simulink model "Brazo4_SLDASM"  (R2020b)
settings: Solver=VariableStepAuto  StartTime=0.0  StopTime=20  RelTol=1e-3
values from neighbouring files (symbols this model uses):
  q = [q 0]    [robotSimulation.m]    (also in robotSimulationWithConstraints.m = [q' 0])
undefined symbols (not defined in the file or in its folder): deg, kg, m, N, rad, s, X, Y, Z
libraries: sm_lib x118, nesl_utility x17, pid_lib x4
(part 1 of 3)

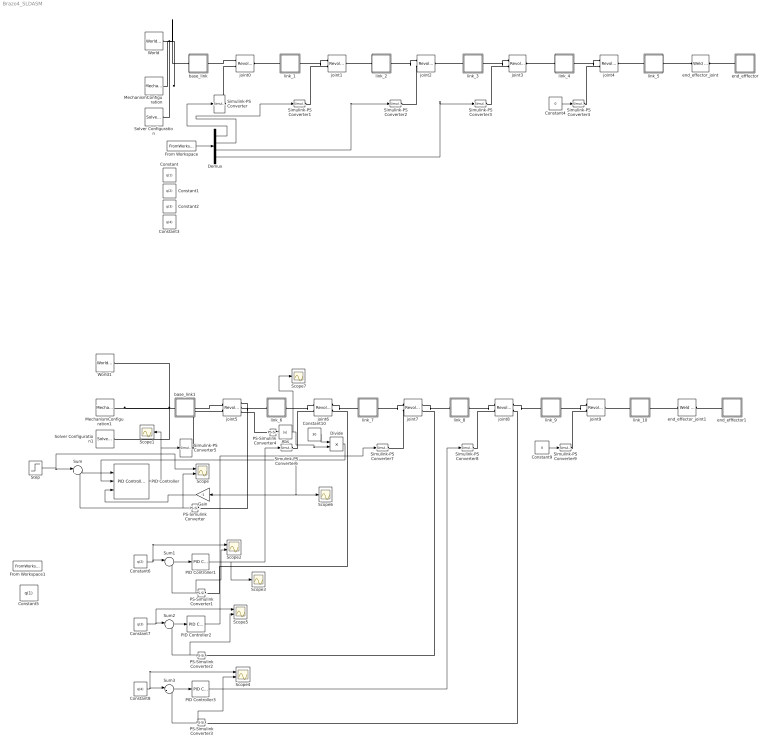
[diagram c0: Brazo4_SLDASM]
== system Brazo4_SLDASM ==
  Abs : Abs
  Constant : Constant  Commented=on  Value=q(1)
  Constant1 : Constant  Commented=on  Value=q(2)
  Constant10 : Constant  Value=30
  Constant2 : Constant  Commented=on  Value=q(3)
  Constant3 : Constant  Commented=on  Value=q(4)
  Constant4 : Constant  Commented=on  Value=0
  Constant5 : Constant  Value=q(1)
  Constant6 : Constant  Value=q(2)
  Constant7 : Constant  Value=q(3)
  Constant8 : Constant  Value=q(4)
  Constant9 : Constant  Value=0
  Demux : Demux  Commented=on
  Divide : Product  Inputs=*/
  From Workspace : FromWorkspace  Commented=on  VariableName=simq
  From Workspace1 : FromWorkspace  VariableName=simq
  Gain : Gain  Gain=-1
  MechanismConfiguration : sm_lib/Utilities/Mechanism Configuration  Commented=on  UniformGravity=Constant  GravityVector=[0 0 -9.80665]  GravityVectorUnits=m/s^2  GravityUnits=m/s^2  LinearizationDelta=0.001  JointModeTransitionNonlinearIterations=2
  MechanismConfiguration1 : sm_lib/Utilities/Mechanism Configuration  UniformGravity=Constant  GravityVector=[0 0 -9.80665]  GravityVectorUnits=m/s^2  GravityUnits=m/s^2  LinearizationDelta=0.001  JointModeTransitionNonlinearIterations=2
  PID Controller : pid_lib/PID Controller  Controller=PD  Form=Parallel  TimeDomain=Continuous-time  UseExternalTs=off  SampleTime=-1  IntegratorMethod=Forward Euler  FilterMethod=Forward Euler  ControllerParametersSource=internal  P=28.6165080032906  I=470.75049682787  D=20.8749963789507  UseFilter=on  N=748.537517356487  TunerSelectOption=Transfer Function Based (PID Tuner App)  InitialConditionSource=internal  InitialConditionForIntegrator=0  InitialConditionForFilter=0  DifferentiatorICPrevScaledInput=0  ExternalReset=none  TrackingMode=off  Kt=1  LimitOutput=on  SatLimitsSource=external  UpperSaturationLimit=inf  LowerSaturationLimit=-inf  LinearizeAsGain=on  AntiWindupMode=none  Kb=1  POutMin=[]  POutMax=[]  IOutMin=[]  IOutMax=[]  DOutMin=[]  DOutMax=[]  NOutMin=[]  NOutMax=[]  SumOutMin=[]  SumOutMax=[]  SaturationOutMin=[]  SaturationOutMax=[]  PParamMin=[]  PParamMax=[]  IParamMin=[]  IParamMax=[]  DParamMin=[]  DParamMax=[]  NParamMin=[]  NParamMax=[]  KbParamMin=[]  KbParamMax=[]  KtParamMin=[]  KtParamMax=[]  KbOutMin=[]  KbOutMax=[]  KtOutMin=[]  KtOutMax=[]  IntegratorOutMin=[]  IntegratorOutMax=[]  FilterOutMin=[]  FilterOutMax=[]  SumI1OutMin=[]  SumI1OutMax=[]  SumI2OutMin=[]  SumI2OutMax=[]  SumI3OutMin=[]  SumI3OutMax=[]  SumI4OutMin=[]  SumI4OutMax=[]  SumDOutMin=[]  SumDOutMax=[]  DifferentiatorOutMin=[]  DifferentiatorOutMax=[]  FilterDiffOutCoefMin=[]  FilterDiffOutCoefMax=[]  ReciprocalOutMin=[]  ReciprocalOutMax=[]  SumDenOutMin=[]  SumDenOutMax=[]  SumNumOutMin=[]  SumNumOutMax=[]  DivideOutMin=[]  DivideOutMax=[]  UdiffTsProdOutMin=[]  UdiffTsProdOutMax=[]  NTsProdOutMin=[]  NTsProdOutMax=[]  UintegralTsProdOutMin=[]  UintegralTsProdOutMax=[]  UngainTsProdOutMin=[]  UngainTsProdOutMax=[]  IntegratorContinuousStateAttributes=''  IntegratorStateMustResolveToSignalObject=off  IntegratorRTWStateStorageClass=Auto  FilterContinuousStateAttributes=''  FilterStateMustResolveToSignalObject=off  FilterRTWStateStorageClass=Auto  ParallelPVariant=InternalParameters  IdealPVariant=Disabled  IVariant=Disabled  DVariant=InternalParameters  IntegratorVariant=Disabled  SatVariant=External  AWVariant=Disabled  PCopyVariant=Disabled  TRVariant=Disabled  FdbkBlocksVariant=Forward  IdealPFdbkVariant=Disabled  SatFdbkVariant=Disabled  DerivativeFilterVariant=ContFilter  NVariant=InternalParameters  NCopyVariant=Disabled  FilterICVariant=InternalICsFilter  IntegratorICVariant=Disabled  ExternalResetVariant=Disabled  TRSumVariant=Passthrough  SumFdbkVariant=Disabled  SumVariant=Sum_PD  TsampFilterVariant=InternalTs  TsampNgainVariant=Passthrough  TsampIntegralVariant=Disabled_SignalSpec  ExternalSaturationOutDataTypeStr=Inherit: Same as second input
  PID Controller1 : pid_lib/PID Controller  Controller=PID  Form=Parallel  TimeDomain=Continuous-time  UseExternalTs=off  SampleTime=-1  IntegratorMethod=Forward Euler  FilterMethod=Forward Euler  ControllerParametersSource=internal  P=623.560595989225  I=560.575968398352  D=154.114613829274  UseFilter=on  N=17610.6564225781  TunerSelectOption=Transfer Function Based (PID Tuner App)  InitialConditionSource=internal  InitialConditionForIntegrator=0  InitialConditionForFilter=0  DifferentiatorICPrevScaledInput=0  ExternalReset=none  TrackingMode=off  Kt=1  LimitOutput=off  SatLimitsSource=internal  UpperSaturationLimit=inf  LowerSaturationLimit=-inf  LinearizeAsGain=on  AntiWindupMode=none  Kb=1  POutMin=[]  POutMax=[]  IOutMin=[]  IOutMax=[]  DOutMin=[]  DOutMax=[]  NOutMin=[]  NOutMax=[]  SumOutMin=[]  SumOutMax=[]  SaturationOutMin=[]  SaturationOutMax=[]  PParamMin=[]  PParamMax=[]  IParamMin=[]  IParamMax=[]  DParamMin=[]  DParamMax=[]  NParamMin=[]  NParamMax=[]  KbParamMin=[]  KbParamMax=[]  KtParamMin=[]  KtParamMax=[]  KbOutMin=[]  KbOutMax=[]  KtOutMin=[]  KtOutMax=[]  IntegratorOutMin=[]  IntegratorOutMax=[]  FilterOutMin=[]  FilterOutMax=[]  SumI1OutMin=[]  SumI1OutMax=[]  SumI2OutMin=[]  SumI2OutMax=[]  SumI3OutMin=[]  SumI3OutMax=[]  SumI4OutMin=[]  SumI4OutMax=[]  SumDOutMin=[]  SumDOutMax=[]  DifferentiatorOutMin=[]  DifferentiatorOutMax=[]  FilterDiffOutCoefMin=[]  FilterDiffOutCoefMax=[]  ReciprocalOutMin=[]  ReciprocalOutMax=[]  SumDenOutMin=[]  SumDenOutMax=[]  SumNumOutMin=[]  SumNumOutMax=[]  DivideOutMin=[]  DivideOutMax=[]  UdiffTsProdOutMin=[]  UdiffTsProdOutMax=[]  NTsProdOutMin=[]  NTsProdOutMax=[]  UintegralTsProdOutMin=[]  UintegralTsProdOutMax=[]  UngainTsProdOutMin=[]  UngainTsProdOutMax=[]  IntegratorContinuousStateAttributes=''  IntegratorStateMustResolveToSignalObject=off  IntegratorRTWStateStorageClass=Auto  FilterContinuousStateAttributes=''  FilterStateMustResolveToSignalObject=off  FilterRTWStateStorageClass=Auto  ParallelPVariant=InternalParameters  IdealPVariant=Disabled  IVariant=InternalParameters  DVariant=InternalParameters  IntegratorVariant=Continuous  SatVariant=Disabled  AWVariant=Passthrough  PCopyVariant=Disabled  TRVariant=Disabled  FdbkBlocksVariant=Forward  IdealPFdbkVariant=Disabled  SatFdbkVariant=Disabled  DerivativeFilterVariant=ContFilter  NVariant=InternalParameters  NCopyVariant=Disabled  FilterICVariant=InternalICsFilter  IntegratorICVariant=InternalICs  ExternalResetVariant=Disabled  TRSumVariant=Passthrough  SumFdbkVariant=Disabled  SumVariant=Sum_PID  TsampFilterVariant=InternalTs  TsampNgainVariant=Passthrough  TsampIntegralVariant=Passthrough  ExternalSaturationOutDataTypeStr=Inherit: Same as second input
  PID Controller2 : pid_lib/PID Controller  Controller=PID  Form=Parallel  TimeDomain=Continuous-time  UseExternalTs=off  SampleTime=-1  IntegratorMethod=Forward Euler  FilterMethod=Forward Euler  ControllerParametersSource=internal  P=25.434810287757  I=25.1632228084928  D=5.35733231569528  UseFilter=on  N=32.4755687633338  TunerSelectOption=Transfer Function Based (PID Tuner App)  InitialConditionSource=internal  InitialConditionForIntegrator=0  InitialConditionForFilter=0  DifferentiatorICPrevScaledInput=0  ExternalReset=none  TrackingMode=off  Kt=1  LimitOutput=off  SatLimitsSource=internal  UpperSaturationLimit=inf  LowerSaturationLimit=-inf  LinearizeAsGain=on  AntiWindupMode=none  Kb=1  POutMin=[]  POutMax=[]  IOutMin=[]  IOutMax=[]  DOutMin=[]  DOutMax=[]  NOutMin=[]  NOutMax=[]  SumOutMin=[]  SumOutMax=[]  SaturationOutMin=[]  SaturationOutMax=[]  PParamMin=[]  PParamMax=[]  IParamMin=[]  IParamMax=[]  DParamMin=[]  DParamMax=[]  NParamMin=[]  NParamMax=[]  KbParamMin=[]  KbParamMax=[]  KtParamMin=[]  KtParamMax=[]  KbOutMin=[]  KbOutMax=[]  KtOutMin=[]  KtOutMax=[]  IntegratorOutMin=[]  IntegratorOutMax=[]  FilterOutMin=[]  FilterOutMax=[]  SumI1OutMin=[]  SumI1OutMax=[]  SumI2OutMin=[]  SumI2OutMax=[]  SumI3OutMin=[]  SumI3OutMax=[]  SumI4OutMin=[]  SumI4OutMax=[]  SumDOutMin=[]  SumDOutMax=[]  DifferentiatorOutMin=[]  DifferentiatorOutMax=[]  FilterDiffOutCoefMin=[]  FilterDiffOutCoefMax=[]  ReciprocalOutMin=[]  ReciprocalOutMax=[]  SumDenOutMin=[]  SumDenOutMax=[]  SumNumOutMin=[]  SumNumOutMax=[]  DivideOutMin=[]  DivideOutMax=[]  UdiffTsProdOutMin=[]  UdiffTsProdOutMax=[]  NTsProdOutMin=[]  NTsProdOutMax=[]  UintegralTsProdOutMin=[]  UintegralTsProdOutMax=[]  UngainTsProdOutMin=[]  UngainTsProdOutMax=[]  IntegratorContinuousStateAttributes=''  IntegratorStateMustResolveToSignalObject=off  IntegratorRTWStateStorageClass=Auto  FilterContinuousStateAttributes=''  FilterStateMustResolveToSignalObject=off  FilterRTWStateStorageClass=Auto  ParallelPVariant=InternalParameters  IdealPVariant=Disabled  IVariant=InternalParameters  DVariant=InternalParameters  IntegratorVariant=Continuous  SatVariant=Disabled  AWVariant=Passthrough  PCopyVariant=Disabled  TRVariant=Disabled  FdbkBlocksVariant=Forward  IdealPFdbkVariant=Disabled  SatFdbkVariant=Disabled  DerivativeFilterVariant=ContFilter  NVariant=InternalParameters  NCopyVariant=Disabled  FilterICVariant=InternalICsFilter  IntegratorICVariant=InternalICs  ExternalResetVariant=Disabled  TRSumVariant=Passthrough  SumFdbkVariant=Disabled  SumVariant=Sum_PID  TsampFilterVariant=InternalTs  TsampNgainVariant=Passthrough  TsampIntegralVariant=Passthrough  ExternalSaturationOutDataTypeStr=Inherit: Same as second input
  PID Controller3 : pid_lib/PID Controller  Controller=PID  Form=Parallel  TimeDomain=Continuous-time  UseExternalTs=off  SampleTime=-1  IntegratorMethod=Forward Euler  FilterMethod=Forward Euler  ControllerParametersSource=internal  P=5.46250972225863  I=4.50861619061035  D=1.47049025552506  UseFilter=on  N=16168.5388750867  TunerSelectOption=Transfer Function Based (PID Tuner App)  InitialConditionSource=internal  InitialConditionForIntegrator=0  InitialConditionForFilter=0  DifferentiatorICPrevScaledInput=0  ExternalReset=none  TrackingMode=off  Kt=1  LimitOutput=off  SatLimitsSource=internal  UpperSaturationLimit=inf  LowerSaturationLimit=-inf  LinearizeAsGain=on  AntiWindupMode=none  Kb=1  POutMin=[]  POutMax=[]  IOutMin=[]  IOutMax=[]  DOutMin=[]  DOutMax=[]  NOutMin=[]  NOutMax=[]  SumOutMin=[]  SumOutMax=[]  SaturationOutMin=[]  SaturationOutMax=[]  PParamMin=[]  PParamMax=[]  IParamMin=[]  IParamMax=[]  DParamMin=[]  DParamMax=[]  NParamMin=[]  NParamMax=[]  KbParamMin=[]  KbParamMax=[]  KtParamMin=[]  KtParamMax=[]  KbOutMin=[]  KbOutMax=[]  KtOutMin=[]  KtOutMax=[]  IntegratorOutMin=[]  IntegratorOutMax=[]  FilterOutMin=[]  FilterOutMax=[]  SumI1OutMin=[]  SumI1OutMax=[]  SumI2OutMin=[]  SumI2OutMax=[]  SumI3OutMin=[]  SumI3OutMax=[]  SumI4OutMin=[]  SumI4OutMax=[]  SumDOutMin=[]  SumDOutMax=[]  DifferentiatorOutMin=[]  DifferentiatorOutMax=[]  FilterDiffOutCoefMin=[]  FilterDiffOutCoefMax=[]  ReciprocalOutMin=[]  ReciprocalOutMax=[]  SumDenOutMin=[]  SumDenOutMax=[]  SumNumOutMin=[]  SumNumOutMax=[]  DivideOutMin=[]  DivideOutMax=[]  UdiffTsProdOutMin=[]  UdiffTsProdOutMax=[]  NTsProdOutMin=[]  NTsProdOutMax=[]  UintegralTsProdOutMin=[]  UintegralTsProdOutMax=[]  UngainTsProdOutMin=[]  UngainTsProdOutMax=[]  IntegratorContinuousStateAttributes=''  IntegratorStateMustResolveToSignalObject=off  IntegratorRTWStateStorageClass=Auto  FilterContinuousStateAttributes=''  FilterStateMustResolveToSignalObject=off  FilterRTWStateStorageClass=Auto  ParallelPVariant=InternalParameters  IdealPVariant=Disabled  IVariant=InternalParameters  DVariant=InternalParameters  IntegratorVariant=Continuous  SatVariant=Disabled  AWVariant=Passthrough  PCopyVariant=Disabled  TRVariant=Disabled  FdbkBlocksVariant=Forward  IdealPFdbkVariant=Disabled  SatFdbkVariant=Disabled  DerivativeFilterVariant=ContFilter  NVariant=InternalParameters  NCopyVariant=Disabled  FilterICVariant=InternalICsFilter  IntegratorICVariant=InternalICs  ExternalResetVariant=Disabled  TRSumVariant=Passthrough  SumFdbkVariant=Disabled  SumVariant=Sum_PID  TsampFilterVariant=InternalTs  TsampNgainVariant=Passthrough  TsampIntegralVariant=Passthrough  ExternalSaturationOutDataTypeStr=Inherit: Same as second input
  PS-Simulink Converter{,1..4} (5 alike) : nesl_utility/PS-Simulink Converter  PhysicalDomain=network_engine_domain  SubClassName=ps_output  LeftPortType=input  RightPortType=output  PseudoPeriodic=off  Frequencies=[]  Unit=inherit  AffineConversion=off
  Scope{,2,4..5} (4 alike) : Scope  NumInputPorts=2
  Scope{1,3,6..7} (4 alike) : Scope
  Simulink-PS Converter{,1..3} (4 alike) : nesl_utility/Simulink-PS Converter  Commented=on  PhysicalDomain=network_engine_domain  SubClassName=ps_input  LeftPortType=input  RightPortType=output  PseudoPeriodic=off  Frequencies=[]  NoiseDistribution=none  NoiseParameters=[]  Unit=1  AffineConversion=off  FilteringAndDerivatives=filter  SimscapeFilterOrder=2  InputFilterTimeConstant=0.001  UdotUserProvided=0
  Simulink-PS Converter4 : nesl_utility/Simulink-PS Converter  Commented=on  PhysicalDomain=network_engine_domain  SubClassName=ps_input  LeftPortType=input  RightPortType=output  PseudoPeriodic=off  Frequencies=[]  NoiseDistribution=none  NoiseParameters=[]  Unit=1  AffineConversion=off  FilteringAndDerivatives=provide  SimscapeFilterOrder=1  InputFilterTimeConstant=0.001  UdotUserProvided=0
  Simulink-PS Converter{5..8} (4 alike) : nesl_utility/Simulink-PS Converter  PhysicalDomain=network_engine_domain  SubClassName=ps_input  LeftPortType=input  RightPortType=output  PseudoPeriodic=off  Frequencies=[]  NoiseDistribution=none  NoiseParameters=[]  Unit=1  AffineConversion=off  FilteringAndDerivatives=filter  SimscapeFilterOrder=2  InputFilterTimeConstant=0.001  UdotUserProvided=0
  Simulink-PS Converter9 : nesl_utility/Simulink-PS Converter  PhysicalDomain=network_engine_domain  SubClassName=ps_input  LeftPortType=input  RightPortType=output  PseudoPeriodic=off  Frequencies=[]  NoiseDistribution=none  NoiseParameters=[]  Unit=1  AffineConversion=off  FilteringAndDerivatives=provide  SimscapeFilterOrder=1  InputFilterTimeConstant=0.001  UdotUserProvided=0
  Solver Configuration : nesl_utility/Solver Configuration  Commented=on  PhysicalDomain=network_engine_domain  SubClassName=solver  LeftPortType=input  RightPortType=generic  Tones=[]  Harmonics=[]  SimulateNoise=off  Profile=off  UseLocalSampling=off  EnableSwitchedLinearOptims=on  FrequencyDomain=off  UseCCode=off  RelTol=0.001  AbsTol=1e-06  MinStep=1e-09  ToWorkspace=off  RevertToSquareIcSolve=off  NumHomotopyIterations=100  PhasorMode=off  PhasorModeNumHarmonics=1  DoDC=off  ResidualTolerance=1e-09  UseLocalSolver=off  LocalSolverChoice=NE_BACKWARD_EULER_ADVANCER  LocalSolverSampleTime=0.001  DoFixedCost=off  MaxNonlinIter=3  MaxModeIter=2  ComputeImpulses=off  ImpulseIterations=2  LinearAlgebra=auto  EquationFormulation=NE_TIME_EF  DelaysMemoryBudget=1024  AutomaticFiltering=on  FilteringTimeConstant=0.001  PartitionStorageMethod=AS_NEEDED  PartitionMemoryBudget=1024  PartitionMethod=ROBUST
  Solver Configuration1 : nesl_utility/Solver Configuration  PhysicalDomain=network_engine_domain  SubClassName=solver  LeftPortType=input  RightPortType=generic  Tones=[]  Harmonics=[]  SimulateNoise=off  Profile=off  UseLocalSampling=off  EnableSwitchedLinearOptims=on  FrequencyDomain=off  UseCCode=off  RelTol=0.001  AbsTol=1e-06  MinStep=1e-09  ToWorkspace=off  RevertToSquareIcSolve=off  NumHomotopyIterations=100  PhasorMode=off  PhasorModeNumHarmonics=1  DoDC=off  ResidualTolerance=1e-09  UseLocalSolver=off  LocalSolverChoice=NE_BACKWARD_EULER_ADVANCER  LocalSolverSampleTime=0.001  DoFixedCost=off  MaxNonlinIter=3  MaxModeIter=2  ComputeImpulses=off  ImpulseIterations=2  LinearAlgebra=auto  EquationFormulation=NE_TIME_EF  DelaysMemoryBudget=1024  AutomaticFiltering=on  FilteringTimeConstant=0.001  PartitionStorageMethod=AS_NEEDED  PartitionMemoryBudget=1024  PartitionMethod=ROBUST
  Step : Step  After=q(1)  SampleTime=0
  Sum{,1..3} (4 alike) : Sum  Inputs=|+-
  World : sm_lib/Frames and Transforms/World Frame  Commented=on
  World1 : sm_lib/Frames and Transforms/World Frame
  base_link : Subsystem  Commented=on
  base_link1 : Subsystem
  end_effector_joint : sm_lib/Joints/Weld Joint  Commented=on  JointMode=Normal  SenseConstraintForce=off  SenseConstraintForceX=off  SenseConstraintForceY=off  SenseConstraintForceZ=off  SenseConstraintTorque=off  SenseConstraintTorqueX=off  SenseConstraintTorqueY=off  SenseConstraintTorqueZ=off  SenseTotalForce=off  SenseTotalForceX=off  SenseTotalForceY=off  SenseTotalForceZ=off  SenseTotalTorque=off  SenseTotalTorqueX=off  SenseTotalTorqueY=off  SenseTotalTorqueZ=off  CompositeWrenchDir=FollowerOnBase  CompositeWrenchFrame=BaseFrame
  end_effector_joint1 : sm_lib/Joints/Weld Joint  JointMode=Normal  SenseConstraintForce=off  SenseConstraintForceX=off  SenseConstraintForceY=off  SenseConstraintForceZ=off  SenseConstraintTorque=off  SenseConstraintTorqueX=off  SenseConstraintTorqueY=off  SenseConstraintTorqueZ=off  SenseTotalForce=off  SenseTotalForceX=off  SenseTotalForceY=off  SenseTotalForceZ=off  SenseTotalTorque=off  SenseTotalTorqueX=off  SenseTotalTorqueY=off  SenseTotalTorqueZ=off  CompositeWrenchDir=FollowerOnBase  CompositeWrenchFrame=BaseFrame
  end_efffector : Subsystem  Commented=on
  end_efffector1 : Subsystem
  joint0 : sm_lib/Joints/Revolute Joint  Commented=on  JointMode=Normal  SenseConstraintForce=off  SenseConstraintForceX=off  SenseConstraintForceY=off  SenseConstraintForceZ=off  SenseConstraintTorque=off  SenseConstraintTorqueX=off  SenseConstraintTorqueY=off  SenseConstraintTorqueZ=off  SenseTotalForce=off  SenseTotalForceX=off  SenseTotalForceY=off  SenseTotalForceZ=off  SenseTotalTorque=off  SenseTotalTorqueX=off  SenseTotalTorqueY=off  SenseTotalTorqueZ=off  CompositeWrenchDir=FollowerOnBase  CompositeWrenchFrame=BaseFrame  EquilibriumPosition=0  EquilibriumPositionUnits=deg  SpringStiffness=0  SpringStiffnessUnits=N*m/deg  DampingCoefficient=0  DampingCoefficientUnits=m^2*kg/s/rad  TorqueActuationMode=ComputedTorque  MotionActuationMode=InputMotion  SensePosition=off  SenseVelocity=off  SenseAcceleration=off  SenseTorqueForce=off  SenseLowerLimitTorqueForce=off  SenseUpperLimitTorqueForce=off  LowerLimitSpecify=on  LowerLimitBound=-2.618  LowerLimitBoundUnits=rad  LowerLimitStiffness=1e4  LowerLimitStiffnessUnits=N*m/deg  LowerLimitDamping=10  LowerLimitDampingUnits=N*m/(deg/s)  LowerLimitTransitionRegionWidth=0.1  LowerLimitTransitionRegionWidthUnits=deg  UpperLimitSpecify=on  UpperLimitBound=2.618  UpperLimitBoundUnits=rad  UpperLimitStiffness=1e4  UpperLimitStiffnessUnits=N*m/deg  UpperLimitDamping=10  UpperLimitDampingUnits=N*m/(deg/s)  UpperLimitTransitionRegionWidth=0.1  UpperLimitTransitionRegionWidthUnits=deg  PositionTargetSpecify=off  PositionTargetPriority=High  PositionTargetValue=0  PositionTargetValueUnits=deg  VelocityTargetSpecify=off  VelocityTargetPriority=High  VelocityTargetValue=0  VelocityTargetValueUnits=deg/s
  joint1 : sm_lib/Joints/Revolute Joint  Commented=on  JointMode=Normal  SenseConstraintForce=off  SenseConstraintForceX=off  SenseConstraintForceY=off  SenseConstraintForceZ=off  SenseConstraintTorque=off  SenseConstraintTorqueX=off  SenseConstraintTorqueY=off  SenseConstraintTorqueZ=off  SenseTotalForce=off  SenseTotalForceX=off  SenseTotalForceY=off  SenseTotalForceZ=off  SenseTotalTorque=off  SenseTotalTorqueX=off  SenseTotalTorqueY=off  SenseTotalTorqueZ=off  CompositeWrenchDir=FollowerOnBase  CompositeWrenchFrame=BaseFrame  EquilibriumPosition=0  EquilibriumPositionUnits=deg  SpringStiffness=0  SpringStiffnessUnits=N*m/deg  DampingCoefficient=0  DampingCoefficientUnits=m^2*kg/s/rad  TorqueActuationMode=ComputedTorque  MotionActuationMode=InputMotion  SensePosition=off  SenseVelocity=off  SenseAcceleration=off  SenseTorqueForce=off  SenseLowerLimitTorqueForce=off  SenseUpperLimitTorqueForce=off  LowerLimitSpecify=on  LowerLimitBound=-1.134  LowerLimitBoundUnits=rad  LowerLimitStiffness=1e4  LowerLimitStiffnessUnits=N*m/deg  LowerLimitDamping=10  LowerLimitDampingUnits=N*m/(deg/s)  LowerLimitTransitionRegionWidth=0.1  LowerLimitTransitionRegionWidthUnits=deg  UpperLimitSpecify=on  UpperLimitBound=1.134  UpperLimitBoundUnits=rad  UpperLimitStiffness=1e4  UpperLimitStiffnessUnits=N*m/deg  UpperLimitDamping=10  UpperLimitDampingUnits=N*m/(deg/s)  UpperLimitTransitionRegionWidth=0.1  UpperLimitTransitionRegionWidthUnits=deg  PositionTargetSpecify=off  PositionTargetPriority=High  PositionTargetValue=0  PositionTargetValueUnits=deg  VelocityTargetSpecify=off  VelocityTargetPriority=High  VelocityTargetValue=0  VelocityTargetValueUnits=deg/s
  joint2 : sm_lib/Joints/Revolute Joint  Commented=on  JointMode=Normal  SenseConstraintForce=off  SenseConstraintForceX=off  SenseConstraintForceY=off  SenseConstraintForceZ=off  SenseConstraintTorque=off  SenseConstraintTorqueX=off  SenseConstraintTorqueY=off  SenseConstraintTorqueZ=off  SenseTotalForce=off  SenseTotalForceX=off  SenseTotalForceY=off  SenseTotalForceZ=off  SenseTotalTorque=off  SenseTotalTorqueX=off  SenseTotalTorqueY=off  SenseTotalTorqueZ=off  CompositeWrenchDir=FollowerOnBase  CompositeWrenchFrame=BaseFrame  EquilibriumPosition=0  EquilibriumPositionUnits=deg  SpringStiffness=0  SpringStiffnessUnits=N*m/deg  DampingCoefficient=0  DampingCoefficientUnits=m^2*kg/s/rad  TorqueActuationMode=ComputedTorque  MotionActuationMode=InputMotion  SensePosition=off  SenseVelocity=off  SenseAcceleration=off  SenseTorqueForce=off  SenseLowerLimitTorqueForce=off  SenseUpperLimitTorqueForce=off  LowerLimitSpecify=on  LowerLimitBound=-0.96  LowerLimitBoundUnits=rad  LowerLimitStiffness=1e4  LowerLimitStiffnessUnits=N*m/deg  LowerLimitDamping=10  LowerLimitDampingUnits=N*m/(deg/s)  LowerLimitTransitionRegionWidth=0.1  LowerLimitTransitionRegionWidthUnits=deg  UpperLimitSpecify=on  UpperLimitBound=0.96  UpperLimitBoundUnits=rad  UpperLimitStiffness=1e4  UpperLimitStiffnessUnits=N*m/deg  UpperLimitDamping=10  UpperLimitDampingUnits=N*m/(deg/s)  UpperLimitTransitionRegionWidth=0.1  UpperLimitTransitionRegionWidthUnits=deg  PositionTargetSpecify=off  PositionTargetPriority=High  PositionTargetValue=0  PositionTargetValueUnits=deg  VelocityTargetSpecify=off  VelocityTargetPriority=High  VelocityTargetValue=0  VelocityTargetValueUnits=deg/s
  joint3 : sm_lib/Joints/Revolute Joint  Commented=on  JointMode=Normal  SenseConstraintForce=off  SenseConstraintForceX=off  SenseConstraintForceY=off  SenseConstraintForceZ=off  SenseConstraintTorque=off  SenseConstraintTorqueX=off  SenseConstraintTorqueY=off  SenseConstraintTorqueZ=off  SenseTotalForce=off  SenseTotalForceX=off  SenseTotalForceY=off  SenseTotalForceZ=off  SenseTotalTorque=off  SenseTotalTorqueX=off  SenseTotalTorqueY=off  SenseTotalTorqueZ=off  CompositeWrenchDir=FollowerOnBase  CompositeWrenchFrame=BaseFrame  EquilibriumPosition=0  EquilibriumPositionUnits=deg  SpringStiffness=0  SpringStiffnessUnits=N*m/deg  DampingCoefficient=0  DampingCoefficientUnits=m^2*kg/s/rad  TorqueActuationMode=ComputedTorque  MotionActuationMode=InputMotion  SensePosition=off  SenseVelocity=off  SenseAcceleration=off  SenseTorqueForce=off  SenseLowerLimitTorqueForce=off  SenseUpperLimitTorqueForce=off  LowerLimitSpecify=on  LowerLimitBound=-1.57  LowerLimitBoundUnits=rad  LowerLimitStiffness=1e4  LowerLimitStiffnessUnits=N*m/deg  LowerLimitDamping=10  LowerLimitDampingUnits=N*m/(deg/s)  LowerLimitTransitionRegionWidth=0.1  LowerLimitTransitionRegionWidthUnits=deg  UpperLimitSpecify=on  UpperLimitBound=1.57  UpperLimitBoundUnits=rad  UpperLimitStiffness=1e4  UpperLimitStiffnessUnits=N*m/deg  UpperLimitDamping=10  UpperLimitDampingUnits=N*m/(deg/s)  UpperLimitTransitionRegionWidth=0.1  UpperLimitTransitionRegionWidthUnits=deg  PositionTargetSpecify=off  PositionTargetPriority=High  PositionTargetValue=0  PositionTargetValueUnits=deg  VelocityTargetSpecify=off  VelocityTargetPriority=High  VelocityTargetValue=0  VelocityTargetValueUnits=deg/s
  joint4 : sm_lib/Joints/Revolute Joint  Commented=on  JointMode=Normal  SenseConstraintForce=off  SenseConstraintForceX=off  SenseConstraintForceY=off  SenseConstraintForceZ=off  SenseConstraintTorque=off  SenseConstraintTorqueX=off  SenseConstraintTorqueY=off  SenseConstraintTorqueZ=off  SenseTotalForce=off  SenseTotalForceX=off  SenseTotalForceY=off  SenseTotalForceZ=off  SenseTotalTorque=off  SenseTotalTorqueX=off  SenseTotalTorqueY=off  SenseTotalTorqueZ=off  CompositeWrenchDir=FollowerOnBase  CompositeWrenchFrame=BaseFrame  EquilibriumPosition=0  EquilibriumPositionUnits=deg  SpringStiffness=0  SpringStiffnessUnits=N*m/deg  DampingCoefficient=0  DampingCoefficientUnits=m^2*kg/s/rad  TorqueActuationMode=ComputedTorque  MotionActuationMode=InputMotion  SensePosition=off  SenseVelocity=off  SenseAcceleration=off  SenseTorqueForce=off  SenseLowerLimitTorqueForce=off  SenseUpperLimitTorqueForce=off  LowerLimitSpecify=on  LowerLimitBound=-3.14  LowerLimitBoundUnits=rad  LowerLimitStiffness=1e4  LowerLimitStiffnessUnits=N*m/deg  LowerLimitDamping=10  LowerLimitDampingUnits=N*m/(deg/s)  LowerLimitTransitionRegionWidth=0.1  LowerLimitTransitionRegionWidthUnits=deg  UpperLimitSpecify=on  UpperLimitBound=3.14  UpperLimitBoundUnits=rad  UpperLimitStiffness=1e4  UpperLimitStiffnessUnits=N*m/deg  UpperLimitDamping=10  UpperLimitDampingUnits=N*m/(deg/s)  UpperLimitTransitionRegionWidth=0.1  UpperLimitTransitionRegionWidthUnits=deg  PositionTargetSpecify=off  PositionTargetPriority=High  PositionTargetValue=0  PositionTargetValueUnits=deg  VelocityTargetSpecify=off  VelocityTargetPriority=High  VelocityTargetValue=0  VelocityTargetValueUnits=deg/s
  joint5 : sm_lib/Joints/Revolute Joint  JointMode=Normal  SenseConstraintForce=off  SenseConstraintForceX=off  SenseConstraintForceY=off  SenseConstraintForceZ=off  SenseConstraintTorque=off  SenseConstraintTorqueX=off  SenseConstraintTorqueY=off  SenseConstraintTorqueZ=off  SenseTotalForce=off  SenseTotalForceX=off  SenseTotalForceY=off  SenseTotalForceZ=off  SenseTotalTorque=off  SenseTotalTorqueX=off  SenseTotalTorqueY=off  SenseTotalTorqueZ=off  CompositeWrenchDir=FollowerOnBase  CompositeWrenchFrame=BaseFrame  EquilibriumPosition=0  EquilibriumPositionUnits=deg  SpringStiffness=0  SpringStiffnessUnits=N*m/deg  DampingCoefficient=0  DampingCoefficientUnits=m^2*kg/s/rad  TorqueActuationMode=InputTorque  MotionActuationMode=ComputedMotion  SensePosition=on  SenseVelocity=on  SenseAcceleration=off  SenseTorqueForce=off  SenseLowerLimitTorqueForce=off  SenseUpperLimitTorqueForce=off  LowerLimitSpecify=on  LowerLimitBound=-2.618  LowerLimitBoundUnits=rad  LowerLimitStiffness=1e10  LowerLimitStiffnessUnits=N*m/deg  LowerLimitDamping=10000  LowerLimitDampingUnits=N*m/(deg/s)  LowerLimitTransitionRegionWidth=0.1  LowerLimitTransitionRegionWidthUnits=deg  UpperLimitSpecify=on  UpperLimitBound=2.618  UpperLimitBoundUnits=rad  UpperLimitStiffness=1e10  UpperLimitStiffnessUnits=N*m/deg  UpperLimitDamping=10000  UpperLimitDampingUnits=N*m/(deg/s)  UpperLimitTransitionRegionWidth=0.1  UpperLimitTransitionRegionWidthUnits=deg  PositionTargetSpecify=off  PositionTargetPriority=High  PositionTargetValue=0  PositionTargetValueUnits=deg  VelocityTargetSpecify=off  VelocityTargetPriority=High  VelocityTargetValue=0  VelocityTargetValueUnits=deg/s
  joint6 : sm_lib/Joints/Revolute Joint  JointMode=Normal  SenseConstraintForce=off  SenseConstraintForceX=off  SenseConstraintForceY=off  SenseConstraintForceZ=off  SenseConstraintTorque=off  SenseConstraintTorqueX=off  SenseConstraintTorqueY=off  SenseConstraintTorqueZ=off  SenseTotalForce=off  SenseTotalForceX=off  SenseTotalForceY=off  SenseTotalForceZ=off  SenseTotalTorque=off  SenseTotalTorqueX=off  SenseTotalTorqueY=off  SenseTotalTorqueZ=off  CompositeWrenchDir=FollowerOnBase  CompositeWrenchFrame=BaseFrame  EquilibriumPosition=0  EquilibriumPositionUnits=deg  SpringStiffness=0  SpringStiffnessUnits=N*m/deg  DampingCoefficient=0  DampingCoefficientUnits=m^2*kg/s/rad  TorqueActuationMode=InputTorque  MotionActuationMode=ComputedMotion  SensePosition=on  SenseVelocity=off  SenseAcceleration=off  SenseTorqueForce=off  SenseLowerLimitTorqueForce=off  SenseUpperLimitTorqueForce=off  LowerLimitSpecify=on  LowerLimitBound=-1.134  LowerLimitBoundUnits=rad  LowerLimitStiffness=1e4  LowerLimitStiffnessUnits=N*m/deg  LowerLimitDamping=10  LowerLimitDampingUnits=N*m/(deg/s)  LowerLimitTransitionRegionWidth=0.1  LowerLimitTransitionRegionWidthUnits=deg  UpperLimitSpecify=on  UpperLimitBound=1.134  UpperLimitBoundUnits=rad  UpperLimitStiffness=1e4  UpperLimitStiffnessUnits=N*m/deg  UpperLimitDamping=10  UpperLimitDampingUnits=N*m/(deg/s)  UpperLimitTransitionRegionWidth=0.1  UpperLimitTransitionRegionWidthUnits=deg  PositionTargetSpecify=off  PositionTargetPriority=High  PositionTargetValue=0  PositionTargetValueUnits=deg  VelocityTargetSpecify=off  VelocityTargetPriority=High  VelocityTargetValue=0  VelocityTargetValueUnits=deg/s
  joint7 : sm_lib/Joints/Revolute Joint  JointMode=Normal  SenseConstraintForce=off  SenseConstraintForceX=off  SenseConstraintForceY=off  SenseConstraintForceZ=off  SenseConstraintTorque=off  SenseConstraintTorqueX=off  SenseConstraintTorqueY=off  SenseConstraintTorqueZ=off  SenseTotalForce=off  SenseTotalForceX=off  SenseTotalForceY=off  SenseTotalForceZ=off  SenseTotalTorque=off  SenseTotalTorqueX=off  SenseTotalTorqueY=off  SenseTotalTorqueZ=off  CompositeWrenchDir=FollowerOnBase  CompositeWrenchFrame=BaseFrame  EquilibriumPosition=0  EquilibriumPositionUnits=deg  SpringStiffness=0  SpringStiffnessUnits=N*m/deg  DampingCoefficient=0  DampingCoefficientUnits=m^2*kg/s/rad  TorqueActuationMode=InputTorque  MotionActuationMode=ComputedMotion  SensePosition=on  SenseVelocity=off  SenseAcceleration=off  SenseTorqueForce=off  SenseLowerLimitTorqueForce=off  SenseUpperLimitTorqueForce=off  LowerLimitSpecify=on  LowerLimitBound=-0.96  LowerLimitBoundUnits=rad  LowerLimitStiffness=1e4  LowerLimitStiffnessUnits=N*m/deg  LowerLimitDamping=10  LowerLimitDampingUnits=N*m/(deg/s)  LowerLimitTransitionRegionWidth=0.1  LowerLimitTransitionRegionWidthUnits=deg  UpperLimitSpecify=on  UpperLimitBound=0.96  UpperLimitBoundUnits=rad  UpperLimitStiffness=1e4  UpperLimitStiffnessUnits=N*m/deg  UpperLimitDamping=10  UpperLimitDampingUnits=N*m/(deg/s)  UpperLimitTransitionRegionWidth=0.1  UpperLimitTransitionRegionWidthUnits=deg  PositionTargetSpecify=off  PositionTargetPriority=High  PositionTargetValue=0  PositionTargetValueUnits=deg  VelocityTargetSpecify=off  VelocityTargetPriority=High  VelocityTargetValue=0  VelocityTargetValueUnits=deg/s
  joint8 : sm_lib/Joints/Revolute Joint  JointMode=Normal  SenseConstraintForce=off  SenseConstraintForceX=off  SenseConstraintForceY=off  SenseConstraintForceZ=off  SenseConstraintTorque=off  SenseConstraintTorqueX=off  SenseConstraintTorqueY=off  SenseConstraintTorqueZ=off  SenseTotalForce=off  SenseTotalForceX=off  SenseTotalForceY=off  SenseTotalForceZ=off  SenseTotalTorque=off  SenseTotalTorqueX=off  SenseTotalTorqueY=off  SenseTotalTorqueZ=off  CompositeWrenchDir=FollowerOnBase  CompositeWrenchFrame=BaseFrame  EquilibriumPosition=0  EquilibriumPositionUnits=deg  SpringStiffness=0  SpringStiffnessUnits=N*m/deg  DampingCoefficient=0  DampingCoefficientUnits=m^2*kg/s/rad  TorqueActuationMode=InputTorque  MotionActuationMode=ComputedMotion  SensePosition=on  SenseVelocity=off  SenseAcceleration=off  SenseTorqueForce=off  SenseLowerLimitTorqueForce=off  SenseUpperLimitTorqueForce=off  LowerLimitSpecify=on  LowerLimitBound=-1.57  LowerLimitBoundUnits=rad  LowerLimitStiffness=1e4  LowerLimitStiffnessUnits=N*m/deg  LowerLimitDamping=10  LowerLimitDampingUnits=N*m/(deg/s)  LowerLimitTransitionRegionWidth=0.1  LowerLimitTransitionRegionWidthUnits=deg  UpperLimitSpecify=on  UpperLimitBound=1.57  UpperLimitBoundUnits=rad  UpperLimitStiffness=1e4  UpperLimitStiffnessUnits=N*m/deg  UpperLimitDamping=10  UpperLimitDampingUnits=N*m/(deg/s)  UpperLimitTransitionRegionWidth=0.1  UpperLimitTransitionRegionWidthUnits=deg  PositionTargetSpecify=off  PositionTargetPriority=High  PositionTargetValue=0  PositionTargetValueUnits=deg  VelocityTargetSpecify=off  VelocityTargetPriority=High  VelocityTargetValue=0  VelocityTargetValueUnits=deg/s
  joint9 : sm_lib/Joints/Revolute Joint  JointMode=Normal  SenseConstraintForce=off  SenseConstraintForceX=off  SenseConstraintForceY=off  SenseConstraintForceZ=off  SenseConstraintTorque=off  SenseConstraintTorqueX=off  SenseConstraintTorqueY=off  SenseConstraintTorqueZ=off  SenseTotalForce=off  SenseTotalForceX=off  SenseTotalForceY=off  SenseTotalForceZ=off  SenseTotalTorque=off  SenseTotalTorqueX=off  SenseTotalTorqueY=off  SenseTotalTorqueZ=off  CompositeWrenchDir=FollowerOnBase  CompositeWrenchFrame=BaseFrame  EquilibriumPosition=0  EquilibriumPositionUnits=deg  SpringStiffness=0  SpringStiffnessUnits=N*m/deg  DampingCoefficient=0  DampingCoefficientUnits=m^2*kg/s/rad  TorqueActuationMode=ComputedTorque  MotionActuationMode=InputMotion  SensePosition=off  SenseVelocity=off  SenseAcceleration=off  SenseTorqueForce=off  SenseLowerLimitTorqueForce=off  SenseUpperLimitTorqueForce=off  LowerLimitSpecify=on  LowerLimitBound=-3.14  LowerLimitBoundUnits=rad  LowerLimitStiffness=1e4  LowerLimitStiffnessUnits=N*m/deg  LowerLimitDamping=10  LowerLimitDampingUnits=N*m/(deg/s)  LowerLimitTransitionRegionWidth=0.1  LowerLimitTransitionRegionWidthUnits=deg  UpperLimitSpecify=on  UpperLimitBound=3.14  UpperLimitBoundUnits=rad  UpperLimitStiffness=1e4  UpperLimitStiffnessUnits=N*m/deg  UpperLimitDamping=10  UpperLimitDampingUnits=N*m/(deg/s)  UpperLimitTransitionRegionWidth=0.1  UpperLimitTransitionRegionWidthUnits=deg  PositionTargetSpecify=off  PositionTargetPriority=High  PositionTargetValue=0  PositionTargetValueUnits=deg  VelocityTargetSpecify=off  VelocityTargetPriority=High  VelocityTargetValue=0  VelocityTargetValueUnits=deg/s
  link_1 : Subsystem  Commented=on
  link_10 : Subsystem
  link_2 : Subsystem  Commented=on
  link_3 : Subsystem  Commented=on
  link_4 : Subsystem  Commented=on
  link_5 : Subsystem  Commented=on
  link_6 : Subsystem
  link_7 : Subsystem
  link_8 : Subsystem
  link_9 : Subsystem
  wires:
  Constant4/1 -> Simulink-PS Converter4/1
  From Workspace/1 -> Demux/1
  Demux/1 -> Simulink-PS Converter/1
  Demux/2 -> Simulink-PS Converter1/1
  Demux/3 -> Simulink-PS Converter2/1
  Demux/4 -> Simulink-PS Converter3/1
  PID Controller3/1 -> Simulink-PS Converter8/1
  PID Controller2/1 -> Simulink-PS Converter7/1
  Constant9/1 -> Simulink-PS Converter9/1
  PID Controller/1 -> Simulink-PS Converter5/1, Scope1/1
  Sum/1 -> PID Controller/1
  PS-Simulink Converter/1 -> Scope/2, Sum/2
  Constant6/1 -> Scope2/1, Sum1/1
  Sum1/1 -> PID Controller1/1
  PS-Simulink Converter1/1 -> Scope2/2, Sum1/2
  Constant7/1 -> Scope5/1, Sum2/1
  Sum2/1 -> PID Controller2/1
  PS-Simulink Converter2/1 -> Scope5/2, Sum2/2
  Constant8/1 -> Scope4/1, Sum3/1
  Sum3/1 -> PID Controller3/1
  PS-Simulink Converter3/1 -> Sum3/2, Scope4/2
  PID Controller1/1 -> Scope3/1, Simulink-PS Converter6/1
  Step/1 -> Sum/1, Scope/1
  PS-Simulink Converter4/1 -> Abs/1
  Abs/1 -> Scope7/1, Divide/2
  Constant10/1 -> Divide/1
  Divide/1 -> Scope6/1, Gain/1, PID Controller/2
  Gain/1 -> PID Controller/3
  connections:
  base_link/RConn1 -- joint0/LConn1
  end_effector_joint/RConn1 -- end_efffector/LConn1
  joint4/RConn1 -- link_5/LConn1
  end_effector_joint/LConn1 -- link_5/RConn1
  World/RConn1 -- MechanismConfiguration/RConn1 -- Solver Configuration/RConn1 -- base_link/LConn1
  joint0/RConn1 -- link_1/LConn1
  joint1/LConn1 -- link_1/RConn1
  joint1/RConn1 -- link_2/LConn1
  joint2/LConn1 -- link_2/RConn1
  joint2/RConn1 -- link_3/LConn1
  joint3/LConn1 -- link_3/RConn1
  joint3/RConn1 -- link_4/LConn1
  joint4/LConn1 -- link_4/RConn1
  Simulink-PS Converter/RConn1 -- joint0/LConn2
  Simulink-PS Converter1/RConn1 -- joint1/LConn2
  joint2/LConn2 -- Simulink-PS Converter2/RConn1
  Simulink-PS Converter3/RConn1 -- joint3/LConn2
  Simulink-PS Converter4/RConn1 -- joint4/LConn2
  base_link1/LConn1 -- World1/RConn1 -- MechanismConfiguration1/RConn1 -- Solver Configuration1/RConn1
  joint8/RConn1 -- link_9/LConn1
  joint8/LConn1 -- link_8/RConn1
  end_effector_joint1/RConn1 -- end_efffector1/LConn1
  joint7/LConn1 -- link_7/RConn1
  joint7/RConn1 -- link_8/LConn1
  joint9/LConn1 -- link_9/RConn1
  Simulink-PS Converter8/RConn1 -- joint8/LConn2
  joint6/RConn1 -- link_7/LConn1
  joint5/RConn1 -- link_6/LConn1
  joint6/LConn1 -- link_6/RConn1
  joint7/LConn2 -- Simulink-PS Converter7/RConn1
  base_link1/RConn1 -- joint5/LConn1
  Simulink-PS Converter6/RConn1 -- joint6/LConn2
  end_effector_joint1/LConn1 -- link_10/RConn1
  joint9/RConn1 -- link_10/LConn1
  Simulink-PS Converter5/RConn1 -- joint5/LConn2
  Simulink-PS Converter9/RConn1 -- joint9/LConn2
  joint5/RConn2 -- PS-Simulink Converter/LConn1
  joint6/RConn2 -- PS-Simulink Converter1/LConn1
  joint7/RConn2 -- PS-Simulink Converter2/LConn1
  joint8/RConn2 -- PS-Simulink Converter3/LConn1
  joint5/RConn3 -- PS-Simulink Converter4/LConn1

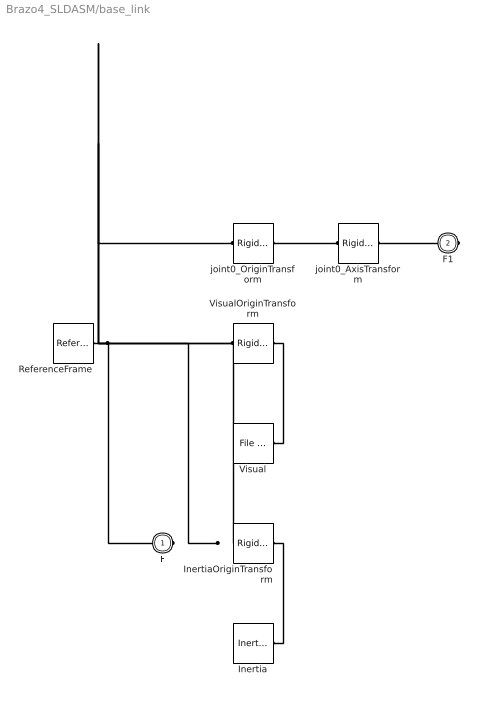
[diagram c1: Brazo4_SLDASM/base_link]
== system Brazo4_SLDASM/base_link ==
  Inertia : sm_lib/Body Elements/Inertia  InertiaType=Custom  Mass=24.751  MassUnits=kg  CenterOfMass=[0, 0, 0]  CenterOfMassUnits=m  MomentsOfInertia=[0.08748, 0.087476, 0.08538900000000001]  MomentsOfInertiaUnits=kg*m^2  ProductsOfInertia=[9.2273e-08, 1.6655e-07, -1.077e-07]  ProductsOfInertiaUnits=kg*m^2  GraphicType=None  MarkerShape=Inertia  MarkerSize=20  GraphicVisPropType=SimpleVisualProperties  GraphicDiffuseColor=[0.5 0.5 0.5]  GraphicSpecularColor=[0.5 0.5 0.5 1.0]  GraphicAmbientColor=[0.15 0.15 0.15 1.0]  GraphicEmissiveColor=[0.0 0.0 0.0 1.0]  GraphicShininess=75  GraphicOpacity=1.0
  InertiaOriginTransform : sm_lib/Frames and Transforms/Rigid Transform  TranslationMethod=Cartesian  TranslationStandardOffset=0  TranslationLengthUnit=m  TranslationStandardAxis=+Z  TranslationCartesianOffset=[-3.389e-08, 1.1139e-06, 0.06952700000000001]  TranslationROffset=0  TranslationROffsetUnits=m  TranslationZOffset=0  TranslationZOffsetUnits=m  TranslationThetaOffset=0  TranslationThetaOffsetUnits=deg  RotationMethod=RotationSequence  RotationAngleUnits=deg  RotationStandardAxis=+Z  RotationAngle=0.0  RotationArbitraryAxis=[0 0 1]  FollAlignAxisA=+X  BaseAlignAxisA=+Y  FollAlignAxisB=+Y  BaseAlignAxisB=+Z  RotationSequenceAxes=BaseAxes  RotationSequence=XYZ  RotationSequenceAngles=[0, 0, 0]  RotationSequenceAnglesUnits=rad  RotationMatrix=[1 0 0; 0 1 0; 0 0 1]
  ReferenceFrame : sm_lib/Frames and Transforms/Reference Frame
  Visual : sm_lib/Body Elements/File Solid  ExtGeomFileName=Brazo4_SLDASM/meshes/base_link.STL  UnitType=Custom  ExtGeomFileUnits=m  StepReaderType=HEX  ExportConvexHullGeometry=off  InertiaType=Custom  Mass=0  MassUnits=kg  CenterOfMass=[0, 0, 0]  CenterOfMassUnits=m  MomentsOfInertia=[0, 0, 0]  MomentsOfInertiaUnits=kg*m^2  ProductsOfInertia=[0, 0, 0]  ProductsOfInertiaUnits=kg*m^2  BasedOnType=DensityFromFile  Density=1000  DensityUnits=kg/m^3  DoExposeReferenceFrame=on  SerializedFrames=<Frames/>  GraphicType=FromGeometry  MarkerShape=Sphere  MarkerSize=10  GraphicVisPropType=SimpleVisualProperties  GraphicDiffuseColor=[0.77647, 0.75686, 0.73725]  GraphicSpecularColor=[0.5 0.5 0.5 1.0]  GraphicAmbientColor=[0.15 0.15 0.15 1.0]  GraphicEmissiveColor=[0.0 0.0 0.0 1.0]  GraphicShininess=75  GraphicOpacity=1
  VisualOriginTransform : sm_lib/Frames and Transforms/Rigid Transform  TranslationMethod=Cartesian  TranslationStandardOffset=0  TranslationLengthUnit=m  TranslationStandardAxis=+Z  TranslationCartesianOffset=[0, 0, 0]  TranslationROffset=0  TranslationROffsetUnits=m  TranslationZOffset=0  TranslationZOffsetUnits=m  TranslationThetaOffset=0  TranslationThetaOffsetUnits=deg  RotationMethod=RotationSequence  RotationAngleUnits=deg  RotationStandardAxis=+Z  RotationAngle=0.0  RotationArbitraryAxis=[0 0 1]  FollAlignAxisA=+X  BaseAlignAxisA=+Y  FollAlignAxisB=+Y  BaseAlignAxisB=+Z  RotationSequenceAxes=BaseAxes  RotationSequence=XYZ  RotationSequenceAngles=[0, 0, 0]  RotationSequenceAnglesUnits=rad  RotationMatrix=[1 0 0; 0 1 0; 0 0 1]
  joint0_AxisTransform : sm_lib/Frames and Transforms/Rigid Transform  TranslationMethod=Cartesian  TranslationStandardOffset=0  TranslationLengthUnit=m  TranslationStandardAxis=+Z  TranslationCartesianOffset=[0, 0, 0]  TranslationROffset=0  TranslationROffsetUnits=m  TranslationZOffset=0  TranslationZOffsetUnits=m  TranslationThetaOffset=0  TranslationThetaOffsetUnits=deg  RotationMethod=ArbitraryAxis  RotationAngleUnits=rad  RotationStandardAxis=+Z  RotationAngle=0  RotationArbitraryAxis=[1, 0, 0]  FollAlignAxisA=+X  BaseAlignAxisA=+Y  FollAlignAxisB=+Y  BaseAlignAxisB=+Z  RotationSequenceAxes=FollowerAxes  RotationSequence=XYX  RotationSequenceAngles=[0 0 0]  RotationSequenceAnglesUnits=deg  RotationMatrix=[1 0 0; 0 1 0; 0 0 1]
  joint0_OriginTransform : sm_lib/Frames and Transforms/Rigid Transform  TranslationMethod=Cartesian  TranslationStandardOffset=0  TranslationLengthUnit=m  TranslationStandardAxis=+Z  TranslationCartesianOffset=[0, 0, 0]  TranslationROffset=0  TranslationROffsetUnits=m  TranslationZOffset=0  TranslationZOffsetUnits=m  TranslationThetaOffset=0  TranslationThetaOffsetUnits=deg  RotationMethod=RotationSequence  RotationAngleUnits=deg  RotationStandardAxis=+Z  RotationAngle=0.0  RotationArbitraryAxis=[0 0 1]  FollAlignAxisA=+X  BaseAlignAxisA=+Y  FollAlignAxisB=+Y  BaseAlignAxisB=+Z  RotationSequenceAxes=BaseAxes  RotationSequence=XYZ  RotationSequenceAngles=[0, 0, 0]  RotationSequenceAnglesUnits=rad  RotationMatrix=[1 0 0; 0 1 0; 0 0 1]
  F : PMIOPort  Side=Left
  F1 : PMIOPort  Port=2  Side=Right
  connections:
  Inertia/RConn1 -- InertiaOriginTransform/RConn1
  ReferenceFrame/RConn1 -- InertiaOriginTransform/LConn1 -- VisualOriginTransform/LConn1 -- joint0_OriginTransform/LConn1 -- F/RConn1
  Visual/RConn1 -- VisualOriginTransform/RConn1
  joint0_AxisTransform/RConn1 -- F1/RConn1
  joint0_AxisTransform/LConn1 -- joint0_OriginTransform/RConn1

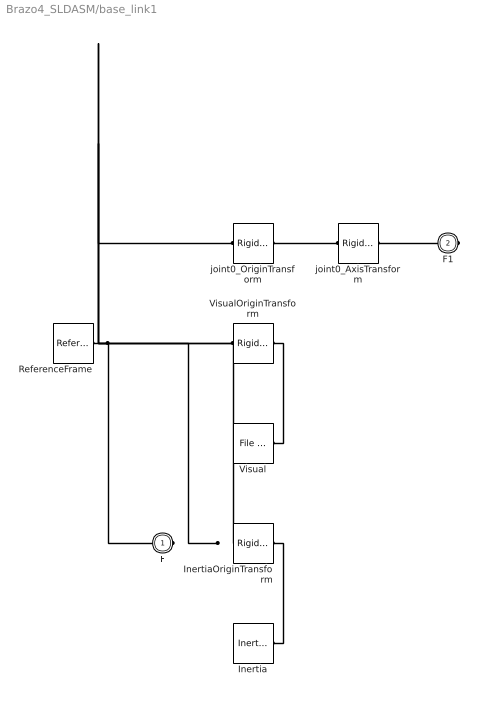
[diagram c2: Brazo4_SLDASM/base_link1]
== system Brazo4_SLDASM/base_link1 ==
  Inertia : sm_lib/Body Elements/Inertia  InertiaType=Custom  Mass=24.751  MassUnits=kg  CenterOfMass=[0, 0, 0]  CenterOfMassUnits=m  MomentsOfInertia=[0.08748, 0.087476, 0.08538900000000001]  MomentsOfInertiaUnits=kg*m^2  ProductsOfInertia=[9.2273e-08, 1.6655e-07, -1.077e-07]  ProductsOfInertiaUnits=kg*m^2  GraphicType=None  MarkerShape=Inertia  MarkerSize=20  GraphicVisPropType=SimpleVisualProperties  GraphicDiffuseColor=[0.5 0.5 0.5]  GraphicSpecularColor=[0.5 0.5 0.5 1.0]  GraphicAmbientColor=[0.15 0.15 0.15 1.0]  GraphicEmissiveColor=[0.0 0.0 0.0 1.0]  GraphicShininess=75  GraphicOpacity=1.0
  InertiaOriginTransform : sm_lib/Frames and Transforms/Rigid Transform  TranslationMethod=Cartesian  TranslationStandardOffset=0  TranslationLengthUnit=m  TranslationStandardAxis=+Z  TranslationCartesianOffset=[-3.389e-08, 1.1139e-06, 0.06952700000000001]  TranslationROffset=0  TranslationROffsetUnits=m  TranslationZOffset=0  TranslationZOffsetUnits=m  TranslationThetaOffset=0  TranslationThetaOffsetUnits=deg  RotationMethod=RotationSequence  RotationAngleUnits=deg  RotationStandardAxis=+Z  RotationAngle=0.0  RotationArbitraryAxis=[0 0 1]  FollAlignAxisA=+X  BaseAlignAxisA=+Y  FollAlignAxisB=+Y  BaseAlignAxisB=+Z  RotationSequenceAxes=BaseAxes  RotationSequence=XYZ  RotationSequenceAngles=[0, 0, 0]  RotationSequenceAnglesUnits=rad  RotationMatrix=[1 0 0; 0 1 0; 0 0 1]
  ReferenceFrame : sm_lib/Frames and Transforms/Reference Frame
  Visual : sm_lib/Body Elements/File Solid  ExtGeomFileName=Brazo4_SLDASM/meshes/base_link.STL  UnitType=Custom  ExtGeomFileUnits=m  StepReaderType=HEX  ExportConvexHullGeometry=off  InertiaType=Custom  Mass=0  MassUnits=kg  CenterOfMass=[0, 0, 0]  CenterOfMassUnits=m  MomentsOfInertia=[0, 0, 0]  MomentsOfInertiaUnits=kg*m^2  ProductsOfInertia=[0, 0, 0]  ProductsOfInertiaUnits=kg*m^2  BasedOnType=DensityFromFile  Density=1000  DensityUnits=kg/m^3  DoExposeReferenceFrame=on  SerializedFrames=<Frames/>  GraphicType=FromGeometry  MarkerShape=Sphere  MarkerSize=10  GraphicVisPropType=SimpleVisualProperties  GraphicDiffuseColor=[0.77647, 0.75686, 0.73725]  GraphicSpecularColor=[0.5 0.5 0.5 1.0]  GraphicAmbientColor=[0.15 0.15 0.15 1.0]  GraphicEmissiveColor=[0.0 0.0 0.0 1.0]  GraphicShininess=75  GraphicOpacity=1
  VisualOriginTransform : sm_lib/Frames and Transforms/Rigid Transform  TranslationMethod=Cartesian  TranslationStandardOffset=0  TranslationLengthUnit=m  TranslationStandardAxis=+Z  TranslationCartesianOffset=[0, 0, 0]  TranslationROffset=0  TranslationROffsetUnits=m  TranslationZOffset=0  TranslationZOffsetUnits=m  TranslationThetaOffset=0  TranslationThetaOffsetUnits=deg  RotationMethod=RotationSequence  RotationAngleUnits=deg  RotationStandardAxis=+Z  RotationAngle=0.0  RotationArbitraryAxis=[0 0 1]  FollAlignAxisA=+X  BaseAlignAxisA=+Y  FollAlignAxisB=+Y  BaseAlignAxisB=+Z  RotationSequenceAxes=BaseAxes  RotationSequence=XYZ  RotationSequenceAngles=[0, 0, 0]  RotationSequenceAnglesUnits=rad  RotationMatrix=[1 0 0; 0 1 0; 0 0 1]
  joint0_AxisTransform : sm_lib/Frames and Transforms/Rigid Transform  TranslationMethod=Cartesian  TranslationStandardOffset=0  TranslationLengthUnit=m  TranslationStandardAxis=+Z  TranslationCartesianOffset=[0, 0, 0]  TranslationROffset=0  TranslationROffsetUnits=m  TranslationZOffset=0  TranslationZOffsetUnits=m  TranslationThetaOffset=0  TranslationThetaOffsetUnits=deg  RotationMethod=ArbitraryAxis  RotationAngleUnits=rad  RotationStandardAxis=+Z  RotationAngle=0  RotationArbitraryAxis=[1, 0, 0]  FollAlignAxisA=+X  BaseAlignAxisA=+Y  FollAlignAxisB=+Y  BaseAlignAxisB=+Z  RotationSequenceAxes=FollowerAxes  RotationSequence=XYX  RotationSequenceAngles=[0 0 0]  RotationSequenceAnglesUnits=deg  RotationMatrix=[1 0 0; 0 1 0; 0 0 1]
  joint0_OriginTransform : sm_lib/Frames and Transforms/Rigid Transform  TranslationMethod=Cartesian  TranslationStandardOffset=0  TranslationLengthUnit=m  TranslationStandardAxis=+Z  TranslationCartesianOffset=[0, 0, 0]  TranslationROffset=0  TranslationROffsetUnits=m  TranslationZOffset=0  TranslationZOffsetUnits=m  TranslationThetaOffset=0  TranslationThetaOffsetUnits=deg  RotationMethod=RotationSequence  RotationAngleUnits=deg  RotationStandardAxis=+Z  RotationAngle=0.0  RotationArbitraryAxis=[0 0 1]  FollAlignAxisA=+X  BaseAlignAxisA=+Y  FollAlignAxisB=+Y  BaseAlignAxisB=+Z  RotationSequenceAxes=BaseAxes  RotationSequence=XYZ  RotationSequenceAngles=[0, 0, 0]  RotationSequenceAnglesUnits=rad  RotationMatrix=[1 0 0; 0 1 0; 0 0 1]
  F : PMIOPort  Side=Left
  F1 : PMIOPort  Port=2  Side=Right
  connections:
  Inertia/RConn1 -- InertiaOriginTransform/RConn1
  ReferenceFrame/RConn1 -- InertiaOriginTransform/LConn1 -- VisualOriginTransform/LConn1 -- joint0_OriginTransform/LConn1 -- F/RConn1
  Visual/RConn1 -- VisualOriginTransform/RConn1
  joint0_AxisTransform/RConn1 -- F1/RConn1
  joint0_AxisTransform/LConn1 -- joint0_OriginTransform/RConn1
